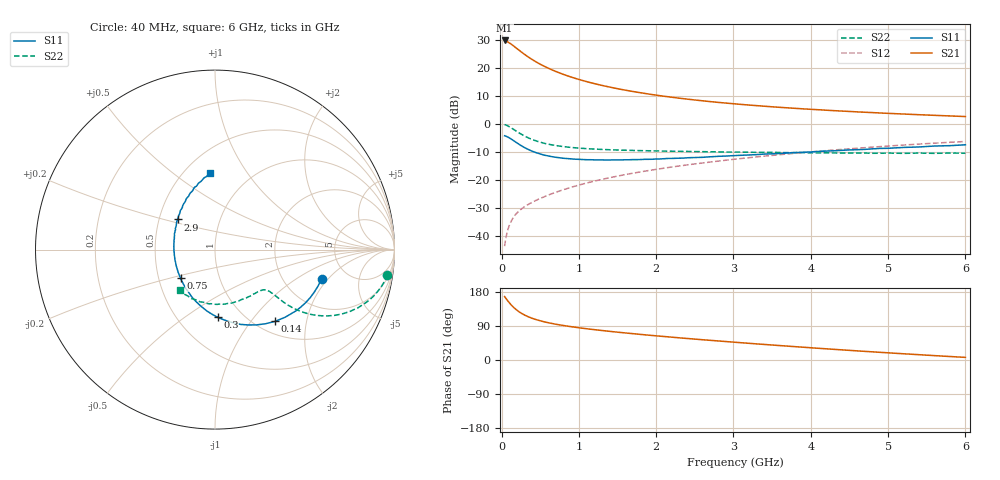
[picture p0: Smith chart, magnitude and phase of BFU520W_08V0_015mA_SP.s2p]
! Filename:  P:\Prog\Test\Noise\ATS_data\Testdata_Net\Run2\BFU520W_APM2013_06_A05_08p0V_015mA_SP_CM01_D.s2p
! Date/Time: Tue 26/Mar/2013 18:01:43
! BFU520W_APM2013_06_A05_08p0V_1to20mA_SP_CM01_Bias7_R.s2p
! MDIF S-parameter v. bias file
! BFU520W_APM2013_06_A05_08p0V_1to20mA_SP_CM01
! Date/time Thu Mar 21 15:28:29 2013
! VAR V_out= 8.0000
! VAR I_out= 14.9950
! VAR V_in= 0.8247
! VAR I_in= 0.1646
! Device data file deembeded for feedlines and parallel
! Original file: \Run2\BFU520W_APM2013_06_A05_08p0V_015mA_SP_CM01_R.s2p
! Feed-files: PR019V01_070313_Feed1.s2p, PR019V01_070313_Feed2.s2p
! Parallel-file: PR019V01_070313_Par.s2p
# MHz S MA R 50
!  Freq-MHz  S11-mag  S11-arg  S21-mag  S21-arg  S12-mag  S12-arg  S22-mag  S22-arg
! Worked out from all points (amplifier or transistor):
!   98 points, 40 MHz to 6 GHz, reference 50 ohm
!   highest |S21| = 29.7 dB at 40 MHz (marker M1)
!   |S21| within 3 dB of that: start of sweep to 204.4 MHz
!   unconditionally stable (mu >= 1): 1.255 GHz to 2.405 GHz
!   at 300 MHz: K = 0.62, MSG = 27.1 dB, |S12| = -29.4 dB
!   at 1.6 GHz: K = 1.01, MAG = 14.4 dB, |S12| = -18.0 dB
!   at 6 GHz: K = 0.88, MSG = 4.4 dB, |S12| = -6.3 dB
!   S11 on the Smith chart (normalised r, x): 40 MHz: 3.23, -1.71; 140 MHz: 1.21, -1.33; 300 MHz: 0.77, -0.68; 750 MHz: 0.65, -0.22; 2.9 GHz: 0.62, +0.23; 6 GHz: 0.66, +0.69
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40  0.6157 -15.4  30.5 167.4  0.006683 83.3  0.9712 -8.3
50  0.6095 -19.3  30.33 164.5  0.008286 82.0  0.9632 -10.3
70  0.5939 -26.8  29.23 159.1  0.01132 78.8  0.9379 -14.2
90  0.5752 -33.9  28.17 153.7  0.01414 76.2  0.9088 -17.7
120  0.5429 -44.0  26.56 146.5  0.01795 73.0  0.8598 -22.2
140  0.5216 -50.0  25.34 142.2  0.02022 71.2  0.8258 -24.7
180  0.4786 -61.2  22.95 134.7  0.0243 68.5  0.7602 -28.8
220  0.4405 -71.1  20.82 128.3  0.02774 67.0  0.7016 -31.7
260  0.4064 -79.6  18.88 123.0  0.03087 66.0  0.6504 -33.8
300  0.378 -87.6  17.18 118.5  0.03379 65.6  0.6072 -35.3
380  0.3339 -100.8  14.44 111.3  0.03923 65.5  0.5397 -36.9
480  0.2981 -114.2  11.95 104.7  0.04587 66.3  0.4827 -37.5
600  0.2702 -127.2  9.871 98.6  0.05385 67.5  0.4371 -37.4
750  0.25 -140.2  8.065 92.7  0.06403 68.6  0.403 -37.3
1050  0.2324 -159.9  5.907 83.8  0.0851 69.9  0.367 -38.1
1500  0.2287 179.4  4.232 73.4  0.1178 69.8  0.3433 -41.6
2050  0.2379 161.7  3.174 62.9  0.1591 68.0  0.3299 -48.1
2900  0.2678 141.1  2.348 48.7  0.2259 63.6  0.3151 -61.9
3100  0.2767 137.0  2.221 45.6  0.2423 62.2  0.3151 -65.3
4100  0.3239 119.8  1.786 30.9  0.3263 54.9  0.3045 -85.4
5200  0.3815 104.0  1.498 16.4  0.4206 45.3  0.2993 -110.4
6000  0.425 93.8  1.352 7.0  0.4867 37.5  0.3004 -130.9
